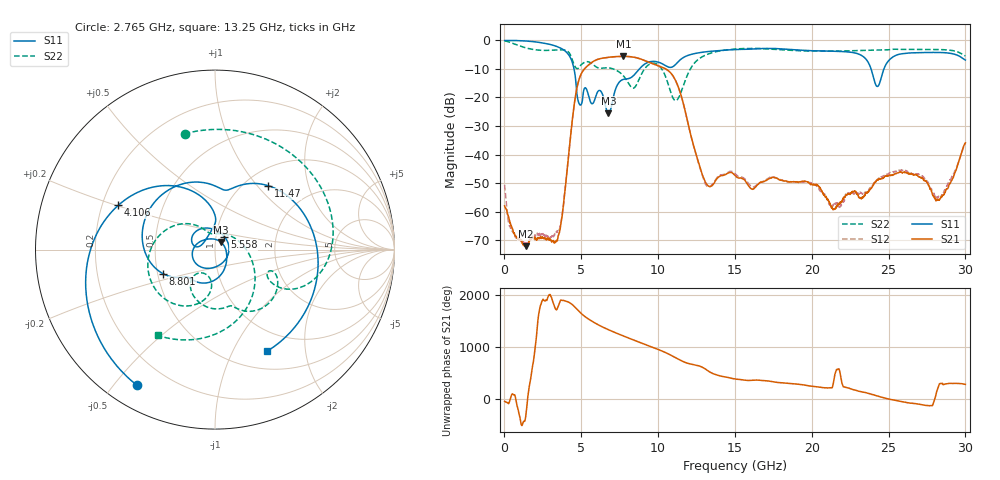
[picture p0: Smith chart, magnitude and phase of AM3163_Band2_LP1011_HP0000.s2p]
!Agilent Technologies,E8364B,MY43040894,A.07.50.67
!Agilent E8364B: A.07.50.67
!Date: Thursday, August 20, 2020 12:03:44
!Correction: S11(Full 2 Port(1,2))
!S21(Full 2 Port(1,2))
!S12(Full 2 Port(1,2))
!S22(Full 2 Port(1,2))
!S2P File: Measurements: S11, S21, S12, S22:
# Hz S  dB  R 50
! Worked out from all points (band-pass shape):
!   3201 points, 10 MHz to 30 GHz, reference 50 ohm
!   highest |S21| = -5.60 dB at 7.742 GHz (marker M1); lowest = -72.1 dB at 1.388 GHz (marker M2)
!   |S21| within 3 dB of the highest: 5.477 GHz to 9.858 GHz (4.381 GHz wide, 57.1 % of centre)
!   lowest |S11| = -25.5 dB at 6.767 GHz (marker M3), VSWR 1.11, Z = 53.2 + j4.5 ohm
!   |S11| at or under -10 dB: 4.528 GHz to 8.785 GHz (4.257 GHz wide, 64 % of centre); 23.86 GHz to 24.7 GHz (839.9 MHz wide, 3.46 % of centre)
!   |S22| runs from -21.1 to -0.2 dB; largest |S21 - S12| = 0.0042
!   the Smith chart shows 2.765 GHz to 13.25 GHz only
!   S11 on the Smith chart (normalised r, x): 2.765 GHz: 0.09, -0.58; 4.106 GHz: 0.27, +0.20; 5.558 GHz: 1.10, +0.16; 8.801 GHz: 0.53, -0.16; 11.47 GHz: 1.27, +1.15; 13.25 GHz: 0.72, -1.37
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1e7  -0.06 -2.9  -57.95 -52.1  -50.61 146.6  -0.18 -8.5
6.660312e8  -0.06 -27.4  -68.10 73.4  -68.02 118.4  -1.31 -77.8
1.387666e9  -0.23 -57.8  -72.06 23.2  -71.02 55.2  -2.62 -147.4
2.765331e9  -1.18 -119.8  -69.67 105.6  -68.60 76.2  -3.52 104.7
3.505709e9  -2.36 -160.0  -68.31 -9.3  -67.03 108.6  -3.32 50.4
4.105509e9  -4.55 155.3  -44.10 77.7  -43.82 77.5  -3.80 -0.7
5.014581e9  -22.26 157.6  -11.55 -155.9  -11.55 -156.2  -8.44 -24.1
5.55815e9  -21.01 53.5  -8.24 84.1  -8.27 83.8  -7.71 -54.7
6.111091e9  -17.71 -140.1  -6.58 -11.3  -6.61 -11.5  -9.66 -73.1
6.767122e9  -25.48 52.4  -5.94 -105.4  -5.97 -105.5  -9.64 -90.8
7.741797e9  -13.68 -120.2  -5.60 133.2  -5.62 133.3  -12.42 -125.0
8.800819e9  -9.91 -155.3  -6.43 8.4  -6.41 8.2  -13.16 -95.6
1.000979e10  -7.63 121.8  -8.89 -128.3  -8.97 -128.5  -8.64 -175.0
1.14718e10  -6.67 50.0  -18.82 20.3  -18.95 20.2  -18.43 36.6
1.325246e10  -3.93 -62.9  -50.92 176.9  -51.33 179.7  -4.81 -123.8
1.5005e10  -3.21 -139.3  -47.28 19.6  -46.63 21.3  -3.04 162.2
1.777908e10  -2.90 96.5  -48.40 -47.1  -48.43 -47.8  -3.20 49.7
2.000958e10  -3.63 -17.1  -50.33 -120.7  -50.12 -119.1  -3.77 -36.5
2.301795e10  -4.73 -140.0  -54.23 145.6  -53.66 142.7  -3.58 -126.5
2.500479e10  -7.11 -131.6  -47.34 -7.4  -46.64 -4.2  -3.29 -176.1
2.821934e10  -4.24 112.0  -55.91 -149.5  -54.97 -151.3  -3.22 99.6
3e10  -6.89 44.6  -35.89 -83.8  -36.14 -82.8  -5.47 46.9
